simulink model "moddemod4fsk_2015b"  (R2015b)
settings: Solver=VariableStepAuto  SolverMode=SingleTasking  StartTime=0.0  StopTime=10.0  RelTol=1e-3
undefined symbols (not defined in the file): DiscIntNeverNeededParam
libraries: dspsrcs4 x2, dspstat3 x1, commrandsrc3 x1

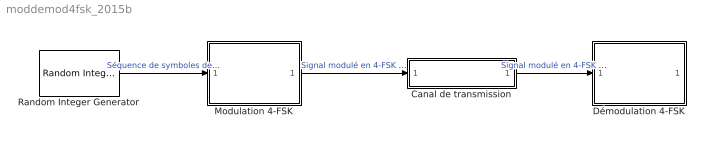
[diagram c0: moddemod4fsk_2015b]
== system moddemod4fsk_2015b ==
  Canal de transmission : Subsystem
  Démodulation 4-FSK : Subsystem
  Modulation 4-FSK : Subsystem
  Random Integer Generator : commrandsrc3/Random Integer Generator  SetSize=4  SeedSource=Auto  Seed=0  SampleTime=1  SamplesPerFrame=1  OutputDataType=double  SimulateUsing=Interpreted execution
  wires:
  Modulation 4-FSK/1(Out1) -> Canal de transmission/1(In1)  "Signal modulé en 4-FSK émis"
  Random Integer Generator/1 -> Modulation 4-FSK/1(In1)  "Séquence de symboles de 2 bits"
  Démodulation 4-FSK/1(Out1) -> ?  "Séquence de symboles de 2 bits démodulé"
  Canal de transmission/1(Out1) -> Démodulation 4-FSK/1(In1)  "Signal modulé en 4-FSK reçu"

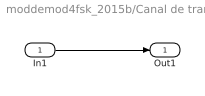
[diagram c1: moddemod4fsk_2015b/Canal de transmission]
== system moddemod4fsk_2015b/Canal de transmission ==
  In1 : Inport
  Out1 : Outport
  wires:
  In1/1 -> Out1/1

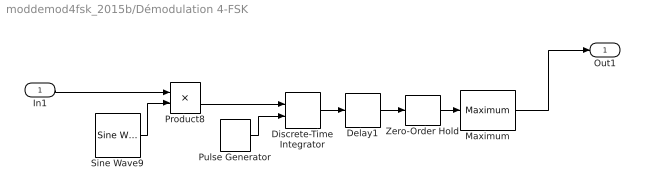
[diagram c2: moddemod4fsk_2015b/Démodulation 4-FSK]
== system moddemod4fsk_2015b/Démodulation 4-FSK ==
  In1 : Inport
  Delay1 : Delay  DelayLength=1
  Discrete-Time Integrator : DiscreteIntegrator  ExternalReset=either  InitialConditionSetting=State (most efficient)  SampleTime=-1  ICPrevOutput=DiscIntNeverNeededParam  ICPrevScaledInput=DiscIntNeverNeededParam
  Maximum : dspstat3/Maximum  operation=maximum  fcn=Index  indexBase=Zero  operateOver=Each row  Dimension=1  InputProcessing=Columns as channels (frame based)  reset=None  roiEnable=off  roiType=Rectangles  roiPortion=Entire ROI  roiOutput=Individual statistics for each ROI  roiFlag=off  roundingMode=Floor  overflowMode=off  accumDataTypeStr=Inherit: Same as product output  accumLastDataTypeStr=Inherit: Same as product output
  Product8 : Product
  Pulse Generator : DiscretePulseGenerator
  Sine Wave9 : dspsrcs4/Sine Wave  Amplitude=1  Frequency=[2:2:8]  Phase=0  SampleMode=Discrete  OutComplex=Real  CompMethod=Trigonometric fcn  TableSize=Speed  SampleTime=1/100  SamplesPerFrame=1  ResetState=Restart at time zero  OutputFrames=off  dataType=double  wordLen=16  udDataType=sfix(16)  fracBitsMode=Best precision  numFracBits=15  OutDataTypeStr=double  LastOutDataTypeStr=double
  Zero-Order Hold : ZeroOrderHold
  Out1 : Outport
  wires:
  Maximum/1 -> Out1/1
  Zero-Order Hold/1 -> Maximum/1
  Pulse Generator/1 -> Discrete-Time Integrator/2
  Delay1/1 -> Zero-Order Hold/1
  In1/1 -> Product8/1
  Product8/1 -> Discrete-Time Integrator/1
  Discrete-Time Integrator/1 -> Delay1/1
  Sine Wave9/1 -> Product8/2

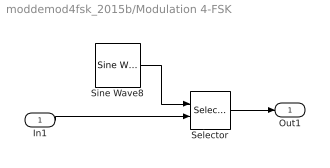
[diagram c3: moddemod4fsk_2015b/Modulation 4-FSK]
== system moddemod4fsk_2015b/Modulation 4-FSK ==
  In1 : Inport
  Selector : Selector  IndexMode=Zero-based  InputPortWidth=4  IndexOptions=Index vector (port)  Indices=[1 3]  OutputSizes=1
  Sine Wave8 : dspsrcs4/Sine Wave  Amplitude=1  Frequency=[2:2:8]  Phase=0  SampleMode=Discrete  OutComplex=Real  CompMethod=Trigonometric fcn  TableSize=Speed  SampleTime=1/100  SamplesPerFrame=1  ResetState=Restart at time zero  OutputFrames=off  dataType=double  wordLen=16  udDataType=sfix(16)  fracBitsMode=Best precision  numFracBits=15  OutDataTypeStr=double  LastOutDataTypeStr=double
  Out1 : Outport
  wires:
  Sine Wave8/1 -> Selector/1
  In1/1 -> Selector/2
  Selector/1 -> Out1/1
